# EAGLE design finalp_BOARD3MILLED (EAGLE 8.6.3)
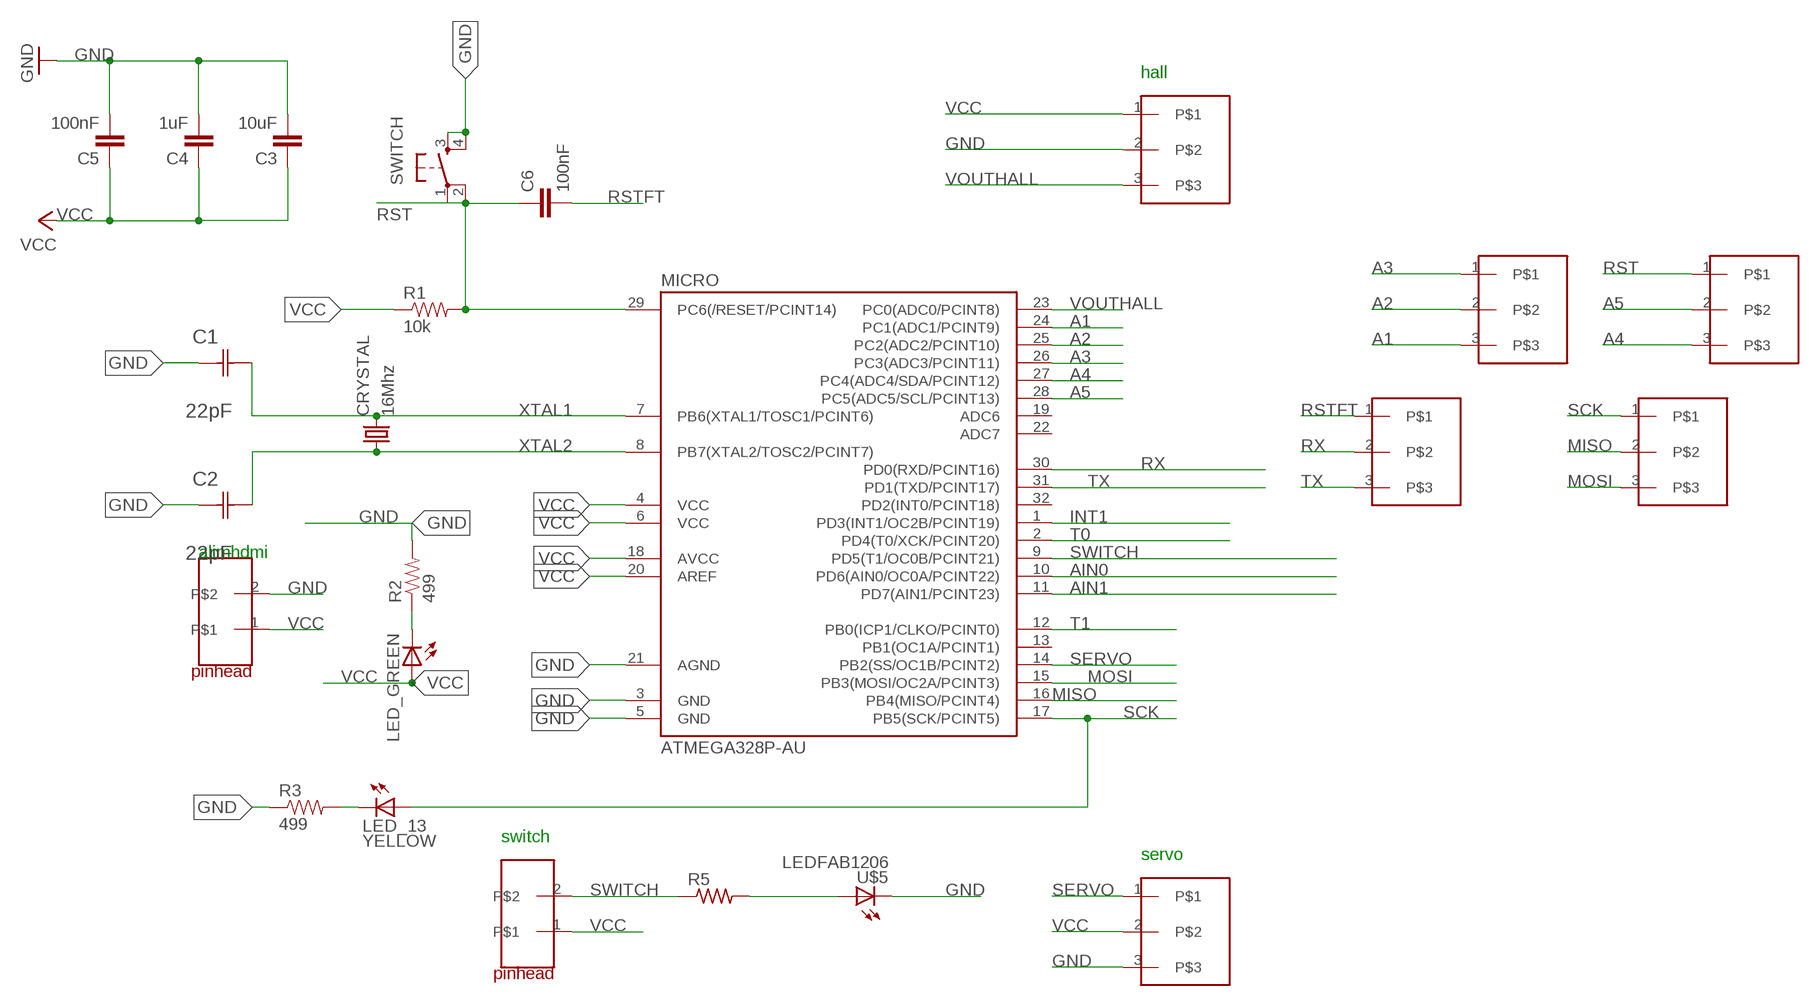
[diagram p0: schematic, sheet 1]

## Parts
C1  22pF  0612ZC225MAT2A  [CAPC3216X178N]
C2  22pF  0612ZC225MAT2A  [CAPC3216X178N]
C3  10uF  CAP1206  [1206]
C4  1uF  CAP1206  [1206]
C5  100nF  CAP1206  [1206]
C6  100nF  CAP1206  [1206]
CRYSTAL  16Mhz  CSM-7X-DU  [CSM-7X-DU]
LED_13  YELLOW  LED1206  [1206]
LED_GREEN  LED1206  [1206]
MICRO  ATMEGA328P-AU  ATMEGA48/88/168-AU  [TQFP32-08]
R1  10k  RESISTOR1206  [1206]
R2  499  RESISTOR1206  [1206]
R3  499  RESISTOR1206  [1206]
R5  RES-US1206FAB  [R1206FAB]
SWITCH  6MM_SWITCH6MM_SWITCH  [6MM_SWITCH]
U$1  PINHEAD3X1BIG  [1X03SMD]
U$2  PINHEAD1X2BIG  [1X02BIG]
U$3  PINHEAD3X1BIG  [1X03SMD]
U$4  PINHEAD1X2BIG  [1X02BIG]
U$5  LEDFAB1206  [LED1206FAB]
U$6  PINHEAD3X1BIG  [1X03SMD]
U$7  PINHEAD3X1BIG  [1X03SMD]
U$8  PINHEAD3X1BIG  [1X03SMD]
U$9  PINHEAD3X1BIG  [1X03SMD]

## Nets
A1: MICRO.24(PC1(ADC1/PCINT9)) U$1.3
A2: MICRO.25(PC2(ADC2/PCINT10)) U$1.2
A3: MICRO.26(PC3(ADC3/PCINT11)) U$1.1
A4: MICRO.27(PC4(ADC4/SDA/PCINT12)) U$9.3
A5: MICRO.28(PC5(ADC5/SCL/PCINT13)) U$9.2
AIN0: MICRO.10(PD6(AIN0/OC0A/PCINT22))
AIN1: MICRO.11(PD7(AIN1/PCINT23))
GND: C1.1(C1) C2.1(C1) C3.2 C4.2 C5.2 MICRO.3(GND) MICRO.5(GND) MICRO.21(AGND) R2.2 R3.1 SWITCH.3(S) SWITCH.4(S1) U$4.2 U$5.2(C) U$6.3 U$7.2
INT1: MICRO.1(PD3(INT1/OC2B/PCINT19))
MISO: MICRO.16(PB4(MISO/PCINT4)) U$8.2
MOSI: MICRO.15(PB3(MOSI/OC2A/PCINT3)) U$8.3
N$2: R5.2 U$5.1(A)
N$26: LED_GREEN.2(C) R2.1
N$27: LED_13.2(C) R3.2
RST: C6.1 MICRO.29(PC6(/RESET/PCINT14)) R1.2 SWITCH.1(P) SWITCH.2(P1) U$9.1
RSTFT: C6.2 U$3.1
RX: MICRO.30(PD0(RXD/PCINT16)) U$3.2
SCK: LED_13.1(A) MICRO.17(PB5(SCK/PCINT5)) U$8.1
SERVO: MICRO.14(PB2(SS/OC1B/PCINT2)) U$6.1
SWITCH: MICRO.9(PD5(T1/OC0B/PCINT21)) R5.1 U$2.2
T0: MICRO.2(PD4(T0/XCK/PCINT20))
T1: MICRO.12(PB0(ICP1/CLKO/PCINT0))
TX: MICRO.31(PD1(TXD/PCINT17)) U$3.3
VCC: C3.1 C4.1 C5.1 LED_GREEN.1(A) MICRO.4(VCC) MICRO.6(VCC) MICRO.18(AVCC) MICRO.20(AREF) R1.1 U$2.1 U$4.1 U$6.2 U$7.1
VOUTHALL: MICRO.23(PC0(ADC0/PCINT8)) U$7.3
XTAL1: C1.2(C2) CRYSTAL.2 MICRO.7(PB6(XTAL1/TOSC1/PCINT6))
XTAL2: C2.2(C2) CRYSTAL.1 MICRO.8(PB7(XTAL2/TOSC2/PCINT7))
Unconnected: MICRO.13(PB1(OC1A/PCINT1)) MICRO.19(ADC6) MICRO.22(ADC7) MICRO.32(PD2(INT0/PCINT18))

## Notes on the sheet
- hall
- alimhdmi
- switch
- servo

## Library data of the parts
C1 C2 = AVX_By_element14_Batch_1:0612ZC225MAT2A: Capacitor 1206; MPN: 0612ZC225MAT2A; OC_FARNELL: -; OC_NEWARK: 12N3209; SUPPLIER: AVX; TOLERANCE: ±20%; VALUE: 2.2µF; VOLTAGERATING: 10V
C3-C6 = 01_SparkFun:CAP: Capacitor
CRYSTAL = 01_FAB_Hello:CSM-7X-DU: SMD CRYSTAL; OC_FARNELL: unknown; OC_NEWARK: unknown
LED_13 LED_GREEN = 01_FAB_Hello:LED
MICRO = atmega8:ATMEGA48/88/168
R1-R3 = 01_SparkFun:RESISTOR: Resistor
R5 = fab:RES-US: Resistor (US Symbol)
SWITCH = 01_FAB_Hello:6MM_SWITCH: OMRON SWITCH
U$1 U$3 U$6-U$9 = fab:PINHEAD3X1BIG
U$2 U$4 = fab:PINHEAD1X2BIG
U$5 = fab:LED: LED

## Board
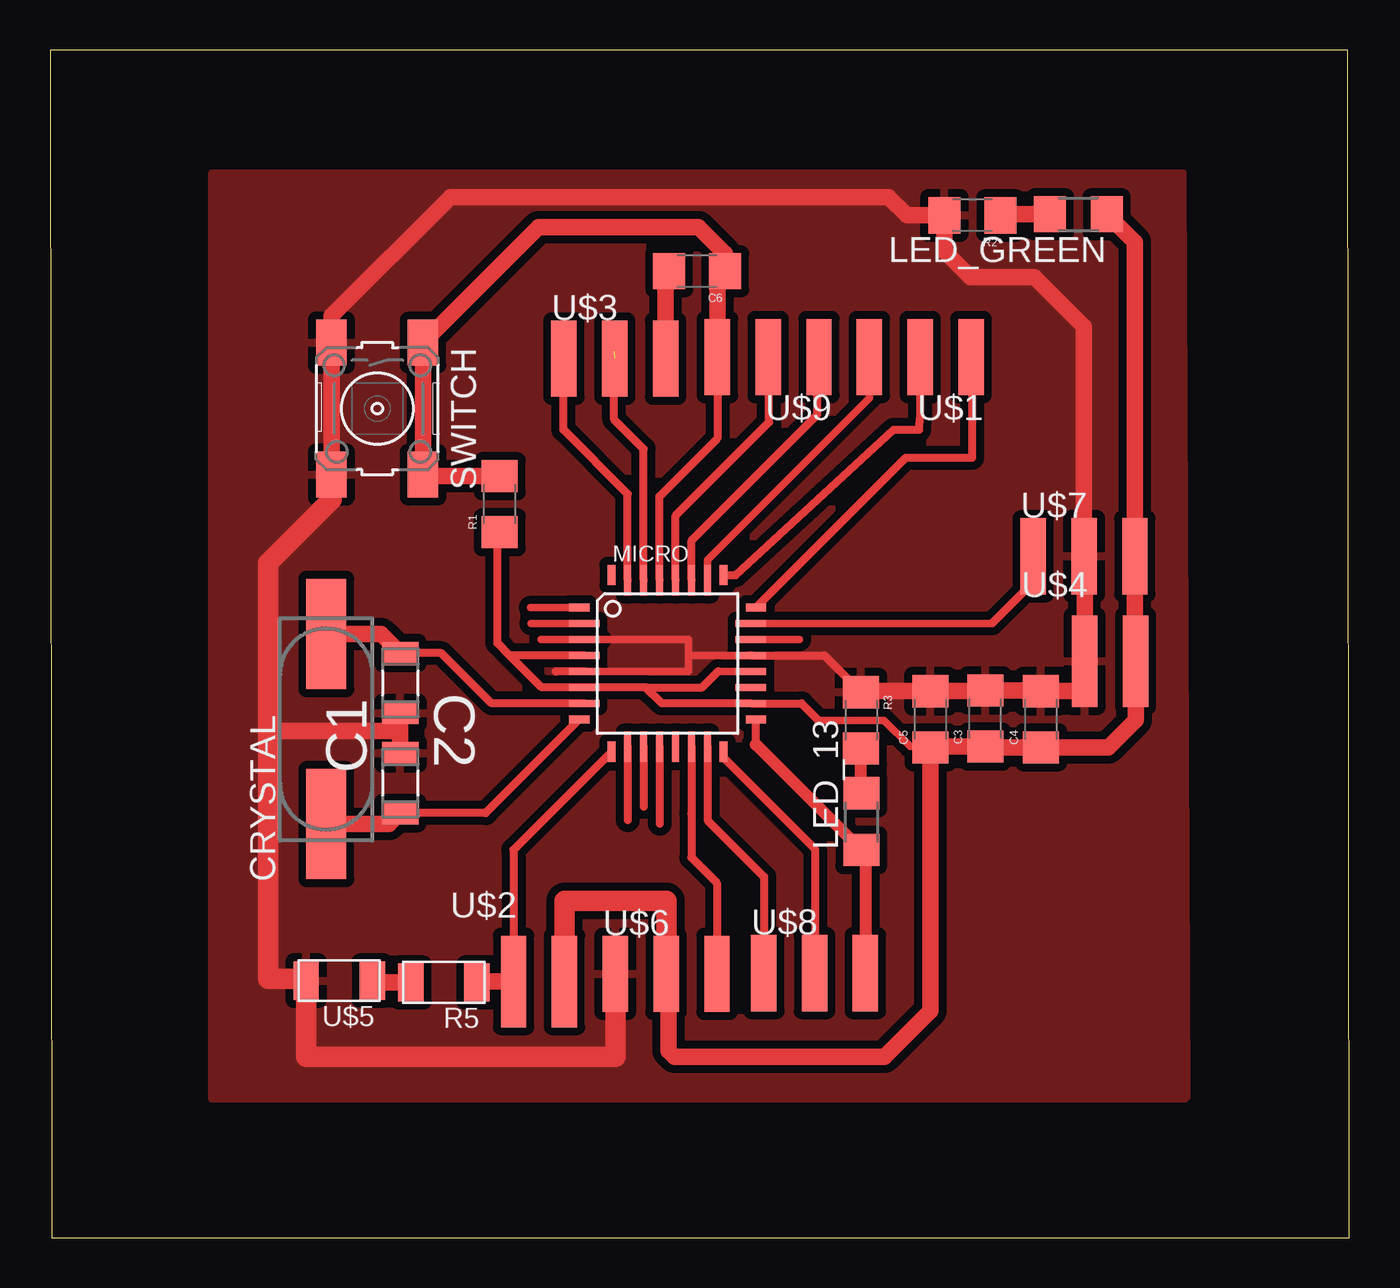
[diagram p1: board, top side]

Size 64.97 x 59.39 mm. Coordinates in mm from the lower left corner, seen from the top.
Outline: 0.08,0 64.97,0 64.89,59.39 0,59.39 0.08,0
Copper layers (1*16): Top 0.035mm / dielectric 1.5mm / Bottom 0.035mm
Design rules "myset *": minimum track width 0.4mm, minimum drill 0.35mm, track to track 0.4mm, track to pad 0.4mm, pad to pad 0.4mm, via to via 0.4mm, smd to smd 0.4mm, copper to edge 40mil, drill to drill 6mil, minimum pad ring 10mil, minimum via ring 8mil, stop-mask expansion 4mil, vias tented up to drill 0mil, thermal gap 16mil

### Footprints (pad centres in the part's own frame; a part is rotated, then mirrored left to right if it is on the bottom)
CAPC3216X178N = smd 1.118 x 1.803: 1 -1.499,0; 2 1.499,0
1206 = smd 1.6 x 1.8: 1 -1.4,0; 2 1.4,0
CSM-7X-DU = smd 5.5 x 2: 1 -4.75,0; 2 4.75,0
1206' = smd 1.6 x 1.803: 1 -1.422,0; 2 1.422,0
TQFP32-08 = smd 1.016 x 0.406: 1 -4.42,2.8; 8 -4.42,-2.8; 17 4.42,-2.8; 24 4.42,2.8 | smd 1.524 x 0.356: 2 -4.166,2; 3 -4.166,1.2; 4 -4.166,0.4; 5 -4.166,-0.4; 6 -4.166,-1.2; 7 -4.166,-2; 18 4.166,-2; 19 4.166,-1.2; 20 4.166,-0.4; 21 4.166,0.4; 22 4.166,1.2; 23 4.166,2 | smd 0.406 x 1.016: 9 -2.8,-4.42; 16 2.8,-4.42; 25 2.8,4.42; 32 -2.8,4.42 | smd 0.356 x 1.524: 10 -2,-4.166; 11 -1.2,-4.166; 12 -0.4,-4.166; 13 0.4,-4.166; 14 1.2,-4.166; 15 2,-4.166; 26 2,4.166; 27 1.2,4.166; 28 0.4,4.166; 29 -0.4,4.166; 30 -1.2,4.166; 31 -2,4.166
R1206FAB = smd 1.27 x 1.905: 1 -1.651,0; 2 1.651,0
6MM_SWITCH = smd 2.286 x 1.524: 1 -3.302,2.286; 2 3.302,2.286; 3 -3.302,-2.286; 4 3.302,-2.286
1X03SMD = smd 3.81 x 1.27: 1 0,6.35; 2 0,3.81; 3 0,1.27
1X02BIG = smd 4.572 x 1.27: 1 0,6.35; 2 0,3.81
LED1206FAB = smd 1.27 x 1.905: 1 -1.651,0; 2 1.651,0

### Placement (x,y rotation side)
C1  17.52,27.74 90 top
C2  17.52,22.74 270 top
C3  46.76,25.96 90 top
C4  49.55,25.93 90 top
C5  44.03,25.93 90 top
C6  32.36,48.33 180 top
CRYSTAL  13.82,25.44 90 top
LED_13  YELLOW  [1206']  40.57,20.81 90 top
LED_GREEN  [1206']  51.42,51.18 180 top
MICRO  30.88,28.72 0 top
R1  22.49,36.68 90 top
R2  46.12,51.12 180 top
R3  40.56,25.88 270 top
R5  19.7,12.77 180 top
SWITCH  16.37,41.46 270 top
U$1  47.32,44.04 90 top
U$2  19.37,12.82 270 top
U$3  24.43,43.96 270 top
U$4  47.93,28.84 270 top
U$5  14.46,12.86 180 top
U$6  27,13.2 270 top
U$7  47.89,34.08 270 top
U$8  34.42,13.24 270 top
U$9  39.72,44.04 90 top

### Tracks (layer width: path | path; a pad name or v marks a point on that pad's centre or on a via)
A1
  Top 0.406: 46.05,42.27 U$1.3 46.12,43.97 46.12,39.01 42.78,39.01 MICRO.24
A2
  Top 0.406: 43.51,42.97 U$1.2 43.51,41.1 43.45,40.4 42.18,40.4 34.28,33.14 MICRO.25
A3
  Top 0.381: MICRO.26 32.88,33.89 40.97,41.98 U$1.1
A4
  Top 0.406: U$9.3 38.37,43.96 38.37,41.17 32.08,34.87 MICRO.27
A5
  Top 0.406: U$9.2 35.96,43.99 35.96,40.79 31.28,36.11 MICRO.28
AIN0
  Top 0.406: MICRO.10 28.88,20.88
AIN1
  Top 0.406: MICRO.11 29.68,21.55
GND
  Top 0.368: 31.92,29.92 31.92,29.12 31.92,28.32 MICRO.5
  Top 0.38: MICRO.21 31.92,29.12 | MICRO.3 31.92,29.92
  Top 0.406: MICRO.21 38.72,29.12 R3.1 | MICRO.5 25.29,28.32 25.29,28.31
  Top 0.813: SWITCH.4 SWITCH.3 14.08,46.1 20.02,52.04 41.92,52.04 42.84,51.12 R2.2 44.72,49.34 46.02,48.04 49.22,48.04 51.7,45.56 U$7.2 51.74,34.04 U$4.2 51.72,28.82 51.72,27.44 51.61,27.33 C4.2 49.52,27.36 C3.2 46.73,27.33 C5.2 40.61,27.33 R3.1 | C1.1 17.52,25.34 | 17.52,25.34 C2.1 | 10.92,25.44 10.92,25.34 17.52,25.34
  Top 1.016: U$6.3 28.27,9.04 12.82,9.04 U$5.2 12.72,12.94 10.92,12.94 10.92,25.44 10.92,33.74 14.08,36.9 SWITCH.4
  pour Top: 8.12,53.24 56.62,53.24 56.82,7.04 56.72,6.94 8.12,6.94
INT1
  Top 0.381: MICRO.1 24.02,31.52 24.02,31.51
MISO
  Top 0.406: MICRO.16 33.68,24.01 38.24,19.45 38.24,13.26 U$8.2
MOSI
  Top 0.406: U$8.3 35.7,13.26 35.7,18.05 32.88,20.88 MICRO.15
N$2
  Top 0.813: R5.2 16.11,12.77 U$5.1
N$3
  Top 0.381: 35.02,29.91 37.48,29.91
N$4
  Top 0.381: 27.47,29.91 24.55,29.91
N$26
  Top 0.813: LED_GREEN.2 47.58,51.18 R2.1
N$27
  Top 0.61: LED_13.2 40.56,22.24 R3.2
RST
  Top 0.406: U$9.1 33.37,39.97 30.47,37.07 30.48,37.07 MICRO.29
  Top 0.813: U$9.1 33.37,47.94 C6.1 33.76,49.2 32.42,50.54 24.43,50.54 SWITCH.1 SWITCH.2 18.73,38.08 R1.2
RSTFT
  Top 0.813: C6.2 30.78,48.15 U$3.1
RX  (1 unrouted)
  Top 0.406: 28.08,44.47 28.21,44.34 28.21,40.91 29.68,39.45 MICRO.30
SCK
  Top 0.406: 35.3,24.66 MICRO.17
  Top 0.61: 35.3,24.66 LED_13.1 40.77,19.19 U$8.1
SERVO
  Top 0.406: U$6.1 33.35,17.74 32.07,19.02 32.07,21.21 32.08,21.22 MICRO.14
SWITCH
  Top 0.406: MICRO.9 23.18,19.4 U$2.2
  Top 0.813: U$2.2 21.35,12.82 R5.1
T0
  Top 0.381: MICRO.2 24.05,30.72
T1
  Top 0.406: MICRO.12 30.48,20.7
TX
  Top 0.406: U$3.3 25.67,43.93 25.67,40.4 28.88,37.2 MICRO.31
VCC  (1 unrouted)
  Top 0.381: 38.37,25.93 38.42,25.87 41.7,25.87 43.01,24.56 44.06,24.56 | 33.4,28.33 33.41,28.32 MICRO.20
  Top 0.406: 22.98,29.12 24.58,27.52 MICRO.6 | 22.98,29.12 22.37,29.74 22.37,34.82 21.9,35.28 | 21.86,35.32 21.9,35.28 | 21.9,35.28 R1.1 | MICRO.4 22.98,29.12 | 29.78,27.53 MICRO.6 | 29.78,27.53 30.59,26.72 MICRO.18 37.58,26.72 38.37,25.93 | 29.78,27.53 32.6,27.53 33.4,28.33
  Top 0.813: LED_GREEN.1 54.24,49.78 U$7.1 54.24,28.88 U$4.1 54.28,25.9 52.91,24.53 C4.1 46.79,24.53 C3.1 44.06,24.56 C5.1 44.03,11.35 41.72,9.04 31.22,9.04 30.92,9.34 30.92,13.09 U$6.2
  Top 1.016: U$2.1 25.72,16.84 30.82,16.84 U$6.2
VOUTHALL
  Top 0.381: MICRO.23 47.1,30.72
  Top 0.406: 47.1,30.72 49.29,32.91 49.16,33.05 U$7.3
XTAL1
  Top 0.406: C1.2 19.56,29.24 22.08,26.72 MICRO.7
  Top 0.813: CRYSTAL.2 16.56,30.19 C1.2
XTAL2
  Top 0.406: MICRO.8 21.78,21.24 C2.2
  Top 0.813: CRYSTAL.1 16.96,20.69 C2.2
